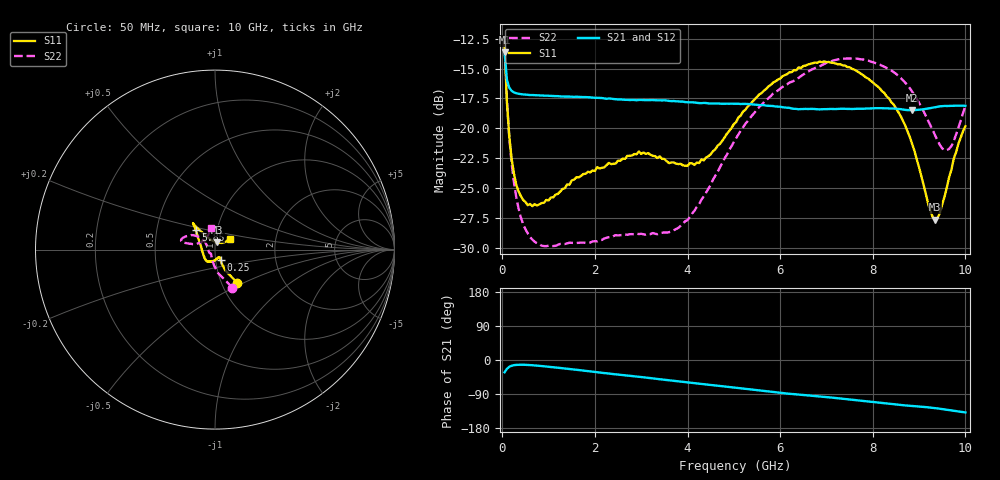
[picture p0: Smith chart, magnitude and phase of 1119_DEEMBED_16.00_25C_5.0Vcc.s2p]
!Hittite Microwave Corp.
!Digital Attenuator/PhaseShifter Rev 1.4.0
!Filename: C:\DATA\DATA\1119_DEEMBED_16.00_25C_5.0Vcc.s2p
!VNA ID: Agilent Technologies,N5224A,MY51441122,A.10.45.03
!Device type:
!2 Port Calibration.
!Temp(C): 25
!Lot Number:
!Serial Number:
!Operator:
!Misc:
!Attenuator:  16.000
# GHZ S DB R 50.0
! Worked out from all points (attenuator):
!   200 points, 50 MHz to 10 GHz, reference 50 ohm
!   highest |S21| = -13.64 dB at 50 MHz (marker M1); lowest = -18.5 dB at 8.85 GHz (marker M2)
!   lowest |S11| = -27.6 dB at 9.35 GHz (marker M3), VSWR 1.09, Z = 50.9 + j4.09 ohm
!   |S11| at or under -10 dB: start of sweep to end of sweep
!   |S22| runs from -29.9 to -12.7 dB; largest |S21 - S12| = 0.00044
!   S11 on the Smith chart (normalised r, x): 50 MHz: 1.18, -0.46; 250 MHz: 1.06, -0.12; 5.85 GHz: 0.79, +0.18; 10 GHz: 1.17, +0.14
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0.05  -13.03 -56.3  -13.64 -32.3  -13.63 -32.3  -12.65 -65.3
0.1  -17.84 -63.7  -15.95 -23.3  -15.94 -23.3  -17.61 -82.6
0.15  -20.64 -64.3  -16.60 -18.0  -16.60 -18.0  -20.74 -92.2
0.25  -23.75 -61.6  -16.99 -13.7  -17.00 -13.7  -24.48 -104.6
0.45  -26.00 -59.5  -17.17 -12.5  -17.17 -12.5  -28.01 -119.4
0.7  -26.35 -64.5  -17.23 -14.3  -17.23 -14.3  -29.50 -129.3
1.75  -23.83 -98.9  -17.39 -27.9  -17.39 -27.9  -29.57 -137.7
2.95  -21.94 -123.7  -17.63 -44.2  -17.64 -44.3  -28.86 -156.8
3.4  -22.35 -139.7  -17.66 -50.7  -17.67 -50.8  -28.80 -170.1
3.8  -23.00 -156.0  -17.75 -56.6  -17.75 -56.7  -28.34 174.2
4.25  -22.91 -177.4  -17.89 -62.7  -17.90 -62.8  -26.36 155.6
5.05  -19.48 148.2  -17.95 -73.2  -17.97 -73.3  -20.83 140.7
5.85  -16.17 134.3  -18.14 -84.6  -18.16 -84.7  -17.09 145.5
6.7  -14.56 130.4  -18.38 -94.4  -18.39 -94.4  -15.05 155.1
7.5  -14.89 130.5  -18.38 -104.1  -18.39 -104.1  -14.16 164.0
8.35  -17.50 127.9  -18.34 -115.2  -18.34 -115.2  -15.05 167.4
8.85  -21.32 121.8  -18.49 -121.3  -18.49 -121.3  -16.93 166.8
9.2  -26.40 99.6  -18.34 -125.0  -18.35 -125.0  -19.41 162.6
9.35  -27.64 75.3  -18.24 -127.0  -18.25 -127.0  -20.63 155.6
9.45  -27.07 57.0  -18.16 -128.7  -18.18 -128.7  -21.40 148.1
9.65  -24.07 39.2  -18.13 -132.2  -18.14 -132.1  -21.72 126.4
10  -19.83 36.9  -18.12 -138.4  -18.12 -138.4  -18.09 99.4
